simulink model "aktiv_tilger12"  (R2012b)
settings: Solver=ode45  StartTime=0.0  StopTime=Tfinal  MaxStep=dt  RelTol=1e-3
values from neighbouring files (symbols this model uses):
  c1 = 20    [aktiv_tilger_1.m]    (also in aktiv_tilger_12.m; aktiv_tilger_2.m = 1; aktiv_tilger_3.m; aktiv_tilger_31.m)
  c2 = 10    [aktiv_tilger_1.m]    (also in aktiv_tilger_12.m; aktiv_tilger_3.m; aktiv_tilger_31.m; beobachter_1.m = 0.5)
  D = 0    [aktiv_tilger_1.m]    (also in aktiv_tilger_12.m; aktiv_tilger_3.m = 2000; aktiv_tilger_31.m; beobachter_1.m)
  Fe1 = 0.5    [aktiv_tilger_1.m]    (also in aktiv_tilger_12.m)
  fsig = 0.01    [aktiv_tilger_1.m]    (also in aktiv_tilger_12.m = 0.1; aktiv_tilger_2.m = 2; aktiv_tilger_3.m = 0.1; diff_filter_1.m = 1)
  I = 2000    [aktiv_tilger_1.m]    (also in aktiv_tilger_12.m; aktiv_tilger_3.m = 0; aktiv_tilger_31.m = 0; fuellstnd_2.m = 0.0225)
  k1 = 100    [aktiv_tilger_1.m]    (also in aktiv_tilger_12.m; aktiv_tilger_2.m = 5; aktiv_tilger_3.m; aktiv_tilger_31.m)
  k2 = 10    [aktiv_tilger_1.m]    (also in aktiv_tilger_12.m; aktiv_tilger_2.m = 10,      c2 = 10; aktiv_tilger_3.m; aktiv_tilger_31.m)
  m1 = 200    [aktiv_tilger_1.m]    (also in aktiv_tilger_12.m; aktiv_tilger_2.m = 100; aktiv_tilger_3.m; aktiv_tilger_31.m)
  m2 = 1    [aktiv_tilger_1.m]    (also in aktiv_tilger_12.m; aktiv_tilger_2.m = 5; aktiv_tilger_3.m; aktiv_tilger_31.m)
  P = 0    [aktiv_tilger_1.m]    (also in aktiv_tilger_12.m; aktiv_tilger_3.m; aktiv_tilger_31.m; fuellstnd_2.m = 0.09)
libraries: simulink x1

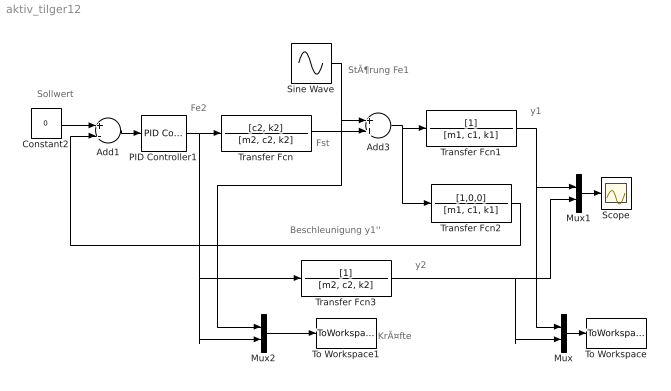
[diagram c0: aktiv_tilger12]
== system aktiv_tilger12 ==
  note: KrÃ¤fte
  note: Sollwert
  note: StÃ¶rung Fe1
  note: y2
  note: Beschleunigung y1''
  note: y1
  note: Fe2
  note: Fst
  Add1 : Sum  Inputs=+-
  Add3 : Sum
  Constant2 : Constant  Value=0
  Mux : Mux  Inputs=2
  Mux1 : Mux  Inputs=2
  Mux2 : Mux  Inputs=2
  PID Controller1 : simulink/Continuous/PID Controller  Controller=PID  TimeDomain=Continuous-time  SampleTime=1  IntegratorMethod=Forward Euler  FilterMethod=Forward Euler  Form=Parallel  P=P  I=I  D=D  N=100  InitialConditionSource=internal  InitialConditionForIntegrator=0  InitialConditionForFilter=0  ExternalReset=none  LimitOutput=off  UpperSaturationLimit=inf  LowerSaturationLimit=-inf  LinearizeAsGain=on  AntiWindupMode=none  Kb=1  TrackingMode=off  Kt=1  PParamMin=[]  PParamMax=[]  IParamMin=[]  IParamMax=[]  DParamMin=[]  DParamMax=[]  NParamMin=[]  NParamMax=[]  KbParamMin=[]  KbParamMax=[]  KtParamMin=[]  KtParamMax=[]  POutMin=[]  POutMax=[]  IOutMin=[]  IOutMax=[]  DOutMin=[]  DOutMax=[]  NOutMin=[]  NOutMax=[]  KbOutMin=[]  KbOutMax=[]  KtOutMin=[]  KtOutMax=[]  IntegratorOutMin=[]  IntegratorOutMax=[]  FilterOutMin=[]  FilterOutMax=[]  SumOutMin=[]  SumOutMax=[]  SumI1OutMin=[]  SumI1OutMax=[]  SumI2OutMin=[]  SumI2OutMax=[]  SumI3OutMin=[]  SumI3OutMax=[]  SumDOutMin=[]  SumDOutMax=[]  SaturationOutMin=[]  SaturationOutMax=[]  IntegratorContinuousStateAttributes=''  IntegratorStateMustResolveToSignalObject=off  IntegratorRTWStateStorageClass=Auto  FilterContinuousStateAttributes=''  FilterStateMustResolveToSignalObject=off  FilterRTWStateStorageClass=Auto
  Scope : Scope
  Sine Wave : Sin  Amplitude=Fe1  Frequency=2*pi*fsig  SampleTime=0
  To Workspace : ToWorkspace  VariableName=y  SampleTime=-1  SaveFormat=Structure With Time
  To Workspace1 : ToWorkspace  VariableName=f  SampleTime=-1  SaveFormat=Structure With Time
  Transfer Fcn : TransferFcn  Numerator=[c2, k2]  Denominator=[m2, c2, k2]
  Transfer Fcn1 : TransferFcn  Denominator=[m1, c1, k1]
  Transfer Fcn2 : TransferFcn  Numerator=[1,0,0]  Denominator=[m1, c1, k1]
  Transfer Fcn3 : TransferFcn  Denominator=[m2, c2, k2]
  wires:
  Add1/1 -> PID Controller1/1
  PID Controller1/1 -> Mux2/2, Transfer Fcn3/1, Transfer Fcn/1
  Constant2/1 -> Add1/1
  Transfer Fcn/1 -> Add3/2
  Add3/1 -> Transfer Fcn2/1, Transfer Fcn1/1
  Transfer Fcn2/1 -> Add1/2
  Transfer Fcn1/1 -> Mux1/1, Mux/1
  Transfer Fcn3/1 -> Mux/2, Mux1/2
  Sine Wave/1 -> Mux2/1, Add3/1
  Mux1/1 -> Scope/1
  Mux/1 -> To Workspace/1
  Mux2/1 -> To Workspace1/1
